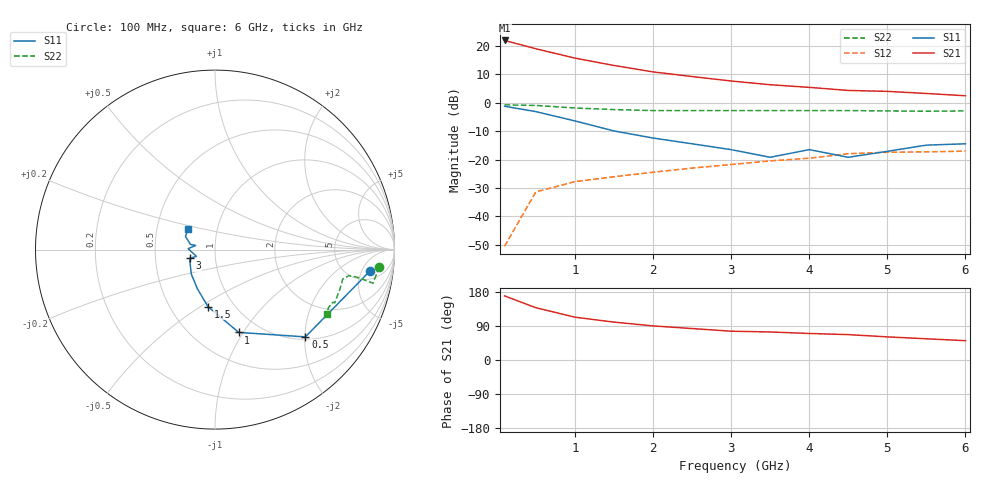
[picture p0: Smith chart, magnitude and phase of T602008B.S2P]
!AT-60200
!S-PARAMETERS at Vce=8V  Ic=5mA.  LAST UPDATED 07-21-92
# ghz s ma r 50
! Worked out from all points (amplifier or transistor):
!   13 points, 100 MHz to 6 GHz, reference 50 ohm
!   highest |S21| = 21.9 dB at 100 MHz (marker M1)
!   |S21| within 3 dB of that: start of sweep to 512.4 MHz
!   unconditionally stable (mu >= 1): 1.7 GHz to end of sweep
!   at 1 GHz: K = 0.70, MSG = 21.7 dB, |S12| = -27.7 dB
!   at 3 GHz: K = 1.16, MAG = 12.3 dB, |S12| = -21.7 dB
!   at 6 GHz: K = 1.20, MAG = 7.1 dB, |S12| = -17.0 dB
!   S11 on the Smith chart (normalised r, x): 100 MHz: 7, -7; 500 MHz: 1.06, -2.01; 1 GHz: 0.80, -0.96; 1.5 GHz: 0.76, -0.54; 3 GHz: 0.75, -0.07; 6 GHz: 0.72, +0.18
0.1  0.87 -8.0  12.51 169.0  0.003 88.0  0.92 -6.0
0.5  0.7 -44.0  8.94 138.0  0.027 72.0  0.9 -12.0
1  0.48 -74.0  6.12 113.0  0.041 65.0  0.81 -11.0
1.5  0.32 -97.0  4.54 100.0  0.05 66.0  0.76 -11.0
2  0.24 -114.0  3.5 90.0  0.06 67.0  0.73 -13.0
2.5  0.19 -134.0  2.9 83.0  0.071 71.0  0.73 -14.0
3  0.15 -161.0  2.42 76.0  0.082 74.0  0.73 -15.0
3.5  0.11 -160.0  2.08 74.0  0.095 75.0  0.73 -18.0
4  0.15 178.0  1.87 70.0  0.106 80.0  0.73 -18.0
4.5  0.11 168.0  1.65 67.0  0.127 76.0  0.73 -24.0
5  0.14 168.0  1.59 61.0  0.135 74.0  0.72 -24.0
5.5  0.18 156.0  1.46 56.0  0.137 73.0  0.71 -27.0
6  0.19 142.0  1.33 51.0  0.141 73.0  0.72 -30.0
